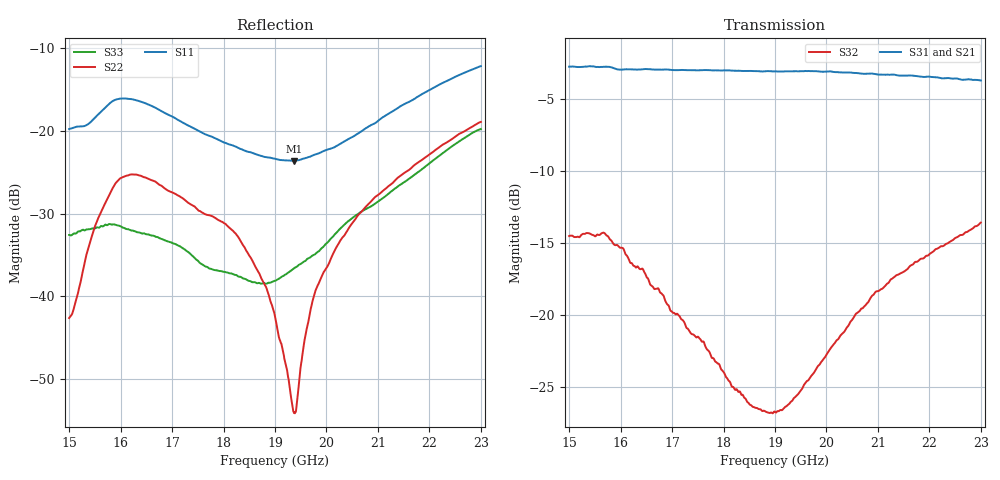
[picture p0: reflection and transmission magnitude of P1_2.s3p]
!The following data was pulled from an Agilent PNA
!This sNp file was generated from the data in the RF Test software
!NOTE:  Smoothing/Math/Corrections applied on any given trace ARE included in the data saved here
# MHz S dB R 50
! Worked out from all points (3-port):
!   1601 points, 15 GHz to 23 GHz, reference 50 ohm
!   strongest paths, dB at 15 GHz, 17 GHz, 19 GHz, 21 GHz, 23 GHz:
!     S31: -2.8, -3.0, -3.1, -3.3, -3.7
!     S21: -3.0, -2.9, -3.1, -3.3, -3.7
!     S32: -14.5, -19.8, -26.7, -18.4, -13.6
!   lowest |S11| = -23.6 dB at 19.37 GHz (marker M1), VSWR 1.14, Z = 49.6 - j6.57 ohm
!   |S11| at or under -10 dB: start of sweep to end of sweep
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15000  -19.78 43.6  -3.05 -167.5  -2.84 -168.7
       -3.03 -167.2  -42.60 160.0  -14.58 152.9
       -2.77 -168.4  -14.53 153.0  -32.57 -138.3
15625  -17.67 49.7  -2.75 -175.4  -2.87 -178.6
       -2.73 -175.6  -29.74 117.3  -14.41 138.5
       -2.79 -178.5  -14.35 138.8  -31.49 136.2
15715  -17.14 47.9  -2.69 -177.1  -2.89 10.5
       -2.68 -176.7  -28.58 110.9  -14.56 134.5
       -2.77 -10.5  -14.45 134.4  -31.33 129.1
15895  -16.26 40.0  -2.70 116.3  -3.04 177.2
       -2.57 10.5  -26.39 93.8  -15.17 128.5
       -2.91 177.0  -15.16 128.1  -31.33 98.2
15970  -16.13 36.4  -2.68 178.5  -3.08 176.3
       -2.59 178.7  -25.87 85.8  -15.30 125.4
       -2.97 176.4  -15.28 125.3  -31.45 86.6
16225  -16.18 24.9  -2.76 174.2  -3.13 173.8
       -2.59 174.2  -25.26 63.1  -16.44 117.6
       -2.96 173.3  -16.45 117.1  -32.03 55.9
19000  -23.37 -69.8  -3.18 137.5  -3.10 137.0
       -3.15 136.9  -42.38 1.9  -26.71 12.3
       -3.10 136.0  -26.74 11.8  -38.11 -93.7
19370  -23.62 -89.7  -3.14 132.1  -3.07 131.5
       -3.13 131.8  -54.06 92.3  -25.73 -13.5
       -3.09 131.0  -25.78 -13.8  -36.59 -123.4
20275  -21.55 -134.4  -3.16 118.6  -3.12 117.7
       -3.16 118.5  -33.19 146.1  -21.39 -62.4
       -3.16 117.6  -21.43 -62.3  -31.76 -169.5
23000  -12.19 157.7  -3.75 78.5  -3.70 78.2
       -3.71 78.8  -18.92 122.9  -13.53 -130.5
       -3.73 78.1  -13.59 -130.8  -19.78 142.4
